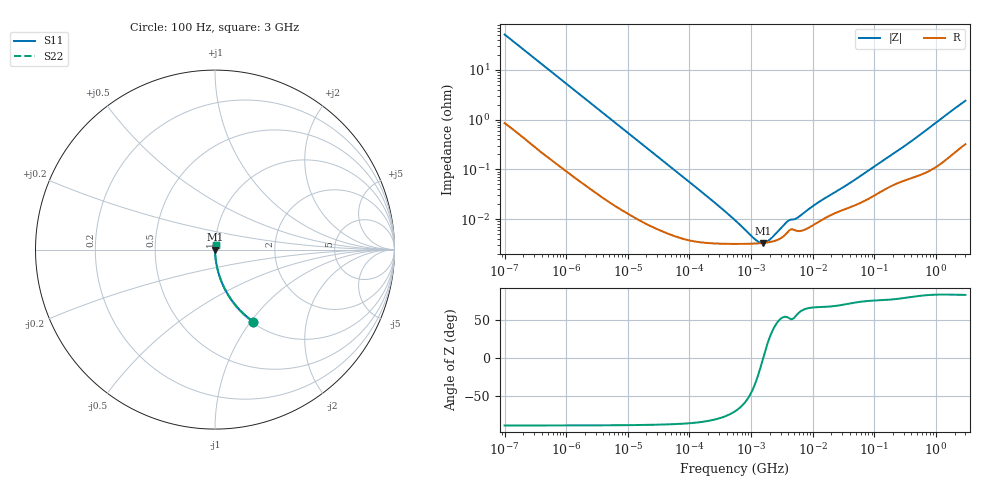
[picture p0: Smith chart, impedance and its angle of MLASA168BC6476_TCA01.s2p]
! MLASA168BC6476_TCA01  S-PARAMETER MODEL  ( Standard Model )
! Model Generated by TAIYO YUDEN Corporation (http://www.ty-top.com)
! Version 1.0
! TAIYO YUDEN Control No. 241206
! Copyright(c) 2024 TAIYO YUDEN CO.,LTD. All Rights Reserved.
! Product Description (link to TY-COMPAS)
! https://ds.yuden.co.jp/TYCOMPAS/or/detail?pn=MLASA168BC6476MTCA01&u=M
! Products Name : Multilayer Ceramic Capacitors
! Characteristics :
!  Capacitance : 47 [uF] , Rated Voltage : 4 [V] , TCC : X6S
!  Case Size : 1.6 x 0.8 / 0.063 x 0.031 [mm/inch] , Thickness : 0.8 / 0.031 [mm/inch]
!  (Conditions: Temperature = 25 [degC] , DC Bias Voltage = 0 [V])
! External Node Assignments :
!  1  o---| |---o  2
! GND o---------o GND
! Frequency Range : 100Hz  -  3GHz  [ 401 STEP ]
# MHZ S RI R 50
! Freq[MHz].  S11 Real  S11 Imag  S21 Real  S21 Imag  S12 Real  S12 Imag  S22 Real  S22 Imag
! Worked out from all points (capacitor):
!   401 points, 100 Hz to 3 GHz, reference 50 ohm
!   read as one part in series: C = 30.7 uF near 109 Hz
!   lowest |Z| = 3.32 mohm at 1.539 MHz (marker M1)
!   series resonance near 1.577 MHz, so ESL is about 330 pH
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0.0001  0.2142 -0.4021  0.7858 0.4021  0.7858 0.4021  0.2142 -0.4021
0.000114  0.1752 -0.3719  0.8248 0.3719  0.8248 0.3719  0.1752 -0.3719
0.000161  0.0987 -0.2899  0.9013 0.2899  0.9013 0.2899  0.0987 -0.2899
0.000269  0.0392 -0.1858  0.9608 0.1858  0.9608 0.1858  0.0392 -0.1858
0.000396  0.0193 -0.1294  0.9807 0.1294  0.9807 0.1294  0.0193 -0.1294
0.000636  0.00817 -0.082  0.9918 0.082  0.9918 0.082  0.00817 -0.082
0.001788  0.00142 -0.0297  0.9986 0.0297  0.9986 0.0297  0.00142 -0.0297
0.005476  0.0003 -0.00984  0.9997 0.00984  0.9997 0.00984  0.0003 -0.00984
0.031977  6.37e-05 -0.00172  0.9999 0.00172  0.9999 0.00172  6.37e-05 -0.00172
0.186741  3.34e-05 -0.000295  1 0.000295  1 0.000295  3.34e-05 -0.000295
0.481374  3.18e-05 -0.000106  1 0.000106  1 0.000106  3.18e-05 -0.000106
0.547723  3.18e-05 -9.01e-05  1 9.01e-05  1 9.01e-05  3.18e-05 -9.01e-05
1.53882  3.32e-05 -1.75e-06  1 1.75e-06  1 1.75e-06  3.32e-05 -1.75e-06
5.135543  6.01e-05 8.06e-05  0.9999 -8.06e-05  0.9999 -8.06e-05  6.01e-05 8.06e-05
5.843389  5.76e-05 9.34e-05  0.9999 -9.34e-05  0.9999 -9.34e-05  5.76e-05 9.34e-05
9.794414  7.38e-05 0.000163  0.9999 -0.000163  0.9999 -0.000163  7.38e-05 0.000163
14.42825  9.85e-05 0.000226  0.9999 -0.000226  0.9999 -0.000226  9.85e-05 0.000226
42.31884  0.000178 0.000527  0.9998 -0.000527  0.9998 -0.000527  0.000178 0.000527
175.1444  0.000445 0.00178  0.9996 -0.00178  0.9996 -0.00178  0.000445 0.00178
414.2403  0.000691 0.00376  0.9993 -0.00376  0.9993 -0.00376  0.000691 0.00376
1950.712  0.00237 0.0161  0.9976 -0.0161  0.9976 -0.0161  0.00237 0.0161
3000  0.00376 0.0237  0.9962 -0.0237  0.9962 -0.0237  0.00376 0.0237
